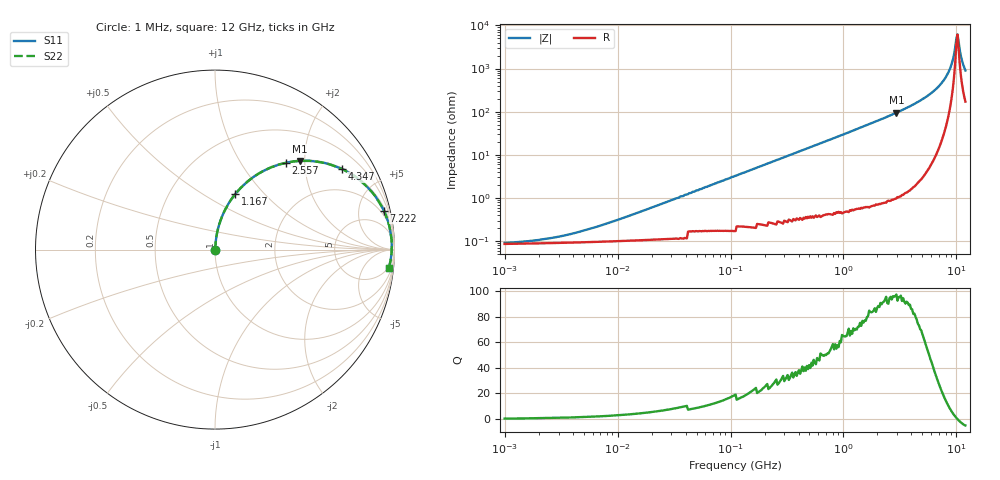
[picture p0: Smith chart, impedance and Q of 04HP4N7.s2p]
# MHz S MA R 50
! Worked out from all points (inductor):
!   408 points, 1 MHz to 12 GHz, reference 50 ohm
!   read as one part in series: L = 4.7 nH near 10.29 MHz
!   highest Q = 95.5 at 2.936 GHz (marker M1), where L = 5.13 nH
!   self-resonance near 9.977 GHz
!   S11 on the Smith chart (normalised r, x): 1 MHz: 1.00, +0.00; 1.167 GHz: 1.01, +0.70; 2.557 GHz: 1.02, +1.61; 4.347 GHz: 1.04, +3.14; 7.222 GHz: 1.36, +8.57; 12 GHz: 4, -18
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1  0.000786 22.0  0.999 -0.0  0.999 -0.0  0.000786 22.0
2.243  0.001033 39.8  0.999 -0.0  0.999 -0.0  0.001033 39.8
4.803  0.001669 58.0  0.999 -0.1  0.999 -0.1  0.001669 58.0
23.071  0.006913 79.5  0.999 -0.4  0.999 -0.4  0.006913 79.5
110.816  0.033 84.7  0.998 -1.9  0.998 -1.9  0.033 84.7
532.275  0.155 79.8  0.984 -8.9  0.984 -8.9  0.155 79.8
1166.549  0.328 70.0  0.94 -19.2  0.94 -19.2  0.328 70.0
1726.976  0.463 61.7  0.881 -27.6  0.881 -27.6  0.463 61.7
2556.642  0.624 50.8  0.775 -38.6  0.775 -38.6  0.624 50.8
2936.332  0.684 46.3  0.723 -43.1  0.723 -43.1  0.684 46.3
4346.99  0.839 32.3  0.534 -57.0  0.534 -57.0  0.839 32.3
5734.022  0.921 21.8  0.372 -67.0  0.372 -67.0  0.921 21.8
7222.457  0.965 13.0  0.225 -74.6  0.225 -74.6  0.965 13.0
8105.835  0.978 8.6  0.15 -77.2  0.15 -77.2  0.978 8.6
8686.912  0.982 6.0  0.105 -77.4  0.105 -77.4  0.982 6.0
9309.645  0.985 3.4  0.061 -73.8  0.061 -73.8  0.985 3.4
9749.407  0.985 1.7  0.032 -61.7  0.032 -61.7  0.985 1.7
9977.019  0.985 0.8  0.02 -41.7  0.02 -41.7  0.985 0.8
10209.94  0.984 -0.1  0.016 4.6  0.016 4.6  0.984 -0.1
10448.31  0.984 -0.9  0.023 44.2  0.023 44.2  0.984 -0.9
11458.72  0.978 -4.4  0.079 71.7  0.079 71.7  0.978 -4.4
12000  0.974 -6.1  0.108 73.0  0.108 73.0  0.974 -6.1
